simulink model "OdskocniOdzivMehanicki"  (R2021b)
settings: Solver=VariableStepAuto  StartTime=0.0  StopTime=3  MaxStep=0.01  RelTol=1e-3
libraries: fl_lib x8, nesl_utility x4

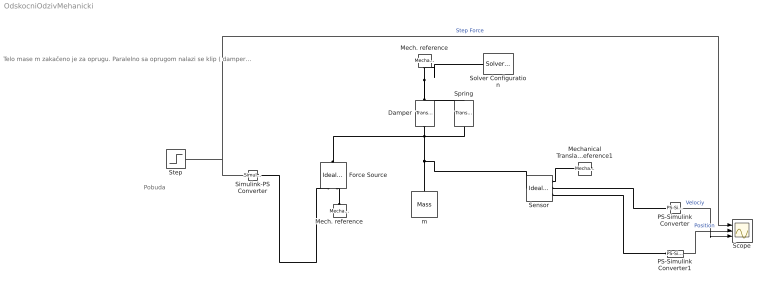
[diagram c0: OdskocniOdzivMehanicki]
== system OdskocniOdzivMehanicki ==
  note: Telo mase m zakačeno je za oprugu. Paralelno sa oprugom nalazi se klip ( damper ) . Klip i opruga su zakačeni za čvrstu tačku ( Mechanical reference ). Pobuda je negativna step sila (npr. gravitacija).
  note: Pobuda
  Damper : fl_lib/Mechanical/Translational Elements/Translational Damper  D=10 N/(m/s)  v_specify=off  v_priority=None  v=0 m/s  v_nominal_specify=off  v_nominal_unit=m/s  v_nominal_value=1  f_specify=off  f_priority=None  f=0 N  f_nominal_specify=off  f_nominal_unit=N  f_nominal_value=1
  Force Source : fl_lib/Mechanical/Mechanical Sources/Ideal Force Source
  Mech. reference : fl_lib/Mechanical/Translational Elements/Mechanical Translational Reference
  Mech. reference : fl_lib/Mechanical/Translational Elements/Mechanical Translational Reference
  Mechanical Translational Reference1 : fl_lib/Mechanical/Translational Elements/Mechanical Translational Reference
  PS-Simulink Converter : nesl_utility/PS-Simulink Converter  PhysicalDomain=network_engine_domain  SubClassName=ps_output  LeftPortType=input  RightPortType=output  PseudoPeriodic=off  Frequencies=[]  Unit=inherit  AffineConversion=off
  PS-Simulink Converter1 : nesl_utility/PS-Simulink Converter  PhysicalDomain=network_engine_domain  SubClassName=ps_output  LeftPortType=input  RightPortType=output  PseudoPeriodic=off  Frequencies=[]  Unit=inherit  AffineConversion=off
  Scope : Scope  NumInputPorts=3
  Sensor : fl_lib/Mechanical/Mechanical Sensors/Ideal Translational Motion Sensor  offset=0 m
  Simulink-PS Converter : nesl_utility/Simulink-PS Converter  PhysicalDomain=network_engine_domain  SubClassName=ps_input  LeftPortType=input  RightPortType=output  PseudoPeriodic=off  Frequencies=[]  NoiseDistribution=none  NoiseParameters=[]  Unit=1  AffineConversion=off  FilteringAndDerivatives=provide  SimscapeFilterOrder=1  InputFilterTimeConstant=0.001  UdotUserProvided=0
  Solver Configuration : nesl_utility/Solver Configuration  PhysicalDomain=network_engine_domain  SubClassName=solver  LeftPortType=input  RightPortType=generic  Tones=[]  Harmonics=[]  SimulateNoise=off  Profile=off  UseLocalSampling=off  EnableSwitchedLinearOptims=on  FrequencyDomain=off  UseCCode=off  RelTol=0.001  AbsTol=1e-06  MinStep=1e-09  ToWorkspace=off  RevertToSquareIcSolve=off  NumHomotopyIterations=100  PhasorMode=off  PhasorModeNumHarmonics=1  DoDC=off  ResidualTolerance=1e-09  UseLocalSolver=off  LocalSolverChoice=NE_BACKWARD_EULER_ADVANCER  LocalSolverSampleTime=0.001  DoFixedCost=off  MaxNonlinIter=3  MaxModeIter=2  ComputeImpulses=off  ImpulseIterations=2  LinearAlgebra=auto  EquationFormulation=NE_TIME_EF  DelaysMemoryBudget=1024  AutomaticFiltering=on  FilteringTimeConstant=0.001  PartitionStorageMethod=AS_NEEDED  PartitionMemoryBudget=1024  PartitionMethod=ROBUST
  Spring : fl_lib/Mechanical/Translational Elements/Translational Spring  spr_rate=2000 N/m  v_specify=off  v_priority=None  v=0 m/s  v_nominal_specify=off  v_nominal_unit=m/s  v_nominal_value=1  f_specify=off  f_priority=None  f=0 N  f_nominal_specify=off  f_nominal_unit=N  f_nominal_value=1  x_specify=off  x_priority=High  x=0 m  x_nominal_specify=off  x_nominal_unit=m  x_nominal_value=1
  Step : Step  After=-10  SampleTime=0
  m : fl_lib/Mechanical/Translational Elements/Mass  mass=1 kg  num_ports=foundation.enum.numPorts2.one  v_specify=off  v_priority=High  v=0 m/s  v_nominal_specify=off  v_nominal_unit=m/s  v_nominal_value=1  f_specify=off  f_priority=None  f=0 N  f_nominal_specify=off  f_nominal_unit=N  f_nominal_value=1
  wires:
  Step/1 -> Simulink-PS Converter/1, Scope/1  "Step Force"
  PS-Simulink Converter1/1 -> Scope/2  "Position"
  PS-Simulink Converter/1 -> Scope/3  "Velociy"
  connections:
  Mech. reference/LConn1 -- Solver Configuration/RConn1 -- Spring/RConn1 -- Damper/RConn1
  Mech. reference/LConn1 -- Force Source/RConn2
  Damper/LConn1 -- Force Source/LConn1 -- Spring/LConn1 -- Sensor/LConn1 -- m/LConn1
  Simulink-PS Converter/RConn1 -- Force Source/RConn1
  Sensor/RConn1 -- Mechanical Translational Reference1/LConn1
  Sensor/RConn2 -- PS-Simulink Converter/LConn1
  Sensor/RConn3 -- PS-Simulink Converter1/LConn1
